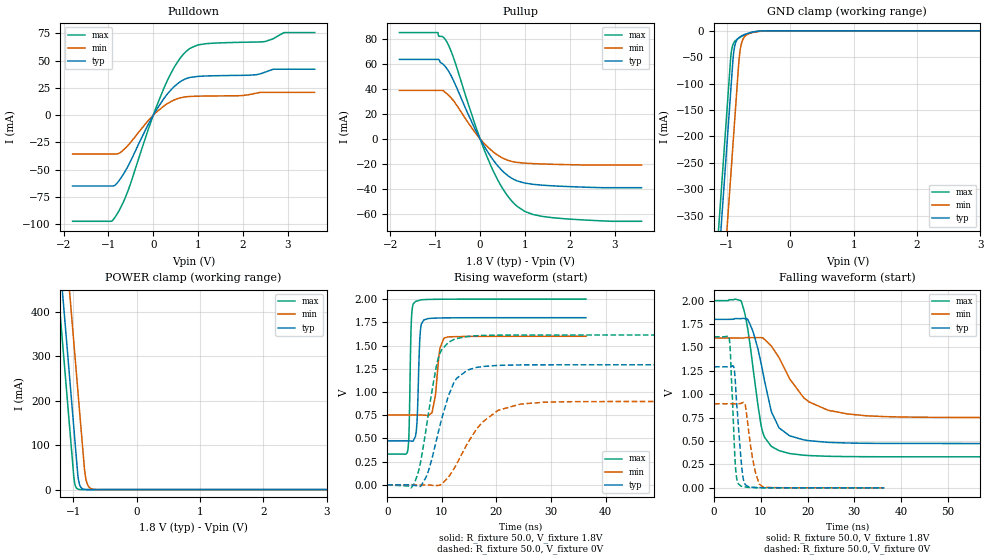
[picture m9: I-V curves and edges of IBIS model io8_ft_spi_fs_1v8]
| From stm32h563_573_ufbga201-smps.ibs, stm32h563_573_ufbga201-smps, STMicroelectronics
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[Model]   io8_ft_spi_fs_1v8
Model_type I/O
Polarity   Non-Inverting
Enable   Active-Low
| CAP_THRESHOLD on pad IOFT is "UDTCAPC" :
| Rising=20.0% of vddiom   Falling=80.0% of vddiom
| C_comp min and max val. don't necessarily correlate with the min and max pvt
| but are the smallest and greatest pad capacitance found.
| var   typ   min   max
C_comp   4.56197pF  4.45395pF  4.75009pF
|C_comp_pullup   2.85165pF  2.67170pF  2.77185pF
|C_comp_pulldown   1.71032pF  1.78225pF  1.97824pF
Vinl = 480.0mV
Vinh = 1.4V
Vmeas = 900.0mV   | Reference voltage for timing measurements
Cref  = 50.0pF   | Timing specification test load capacitance value
Rref  = 100.0MOhm   | Timing specification test load resistance value
Vref  = 900.0mV   | Timing specification test load voltage
[Model Spec]
| TIME_THRESHOLD on pin ZIV11 is "CMOS" :
| Rising=40.0% of vdd   Falling=60.0% of vdd
Vinl 703.80000mV 631.80000mV 784.80000mV
Vinh 1.06220V 937.20000mV 1.16620V
| variable   typ   min   max
[Temperature Range] 25.0 125.0 -40.0
| variable   typ   min   max
[Voltage Range] 1.8V 1.6V 2.0V
| variable   typ   min   max
[POWER Clamp Reference] 1.8V 1.6V 2.0V
| variable   typ   min   max
[GND Clamp Reference] 0V 0V 0V
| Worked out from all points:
|   slope of the pulldown table from 0 to 0.27 V, typ, clamps not added: 15.8 ohm
|   slope of the pullup table from 0 to 0.27 V, typ, clamps not added: 17.1 ohm
|   GND clamp passes 1 mA (typ) near -0.52 V on its own axis
|   POWER clamp passes 1 mA (typ) near -0.84 V on its own axis
|   rising waveform, R_fixture 50.0, V_fixture 1.8V: 20-80 % time 436ps typ, 865ps min, 327ps max; typ from 0.474 V to 1.8 V
|   falling waveform, R_fixture 50.0, V_fixture 1.8V: 20-80 % time 3.87ns typ, 6.87ns min, 2.77ns max; typ from 1.8 V to 0.474 V
|   rising waveform, R_fixture 50.0, V_fixture 0V: 20-80 % time 3.66ns typ, 6.11ns min, 2.71ns max; typ from 0 V to 1.29 V
|   falling waveform, R_fixture 50.0, V_fixture 0V: 20-80 % time 1.19ns typ, 1.67ns min, 840ps max; typ from 1.29 V to 0 V
[POWER Clamp]
-1.8V     1.518A     1.709A     1.407A
-1.23V    548.8mA    740.2mA    437.5mA
-1.16V    429.8mA    621.2mA    318.5mA
-1.05V    242.8mA    434.2mA    131.5mA
-980mV    123.8mA    315.2mA    17.95mA
-930mV    38.81mA    230.2mA    1.49mA
-910mV    17.82mA    196.2mA    550.8uA
-890mV    8.18mA     162.2mA    203.5uA
-810mV    363.5uA    33.6mA     3.797uA
-770mV    76.62uA    10.47mA    518.8nA
-710mV    7.417uA    1.822mA    26.38nA
3.6V      0A         0A         0A
[GND Clamp]
-1.8V     -1.581A    -1.742A    -1.516A
-1.24V    -628.8mA   -789.9mA   -564.1mA
-1.05V    -305.8mA   -466.9mA   -241.1mA
-940mV    -118.8mA   -279.9mA   -54.1mA
-930mV    -101.8mA   -262.9mA   -41.86mA
-900mV    -51.51mA   -211.9mA   -25.34mA
-880mV    -32.22mA   -177.9mA   -21mA
-810mV    -13.02mA   -59.5mA    -13.82mA
-770mV    -9.8mA     -24.99mA   -11mA
-680mV    -5.275mA   -7.288mA   -5.917mA
-400mV    -107uA     -349.1uA   -42.51uA
3.6V      5.392nA    968.2nA    261.3pA
| variable   typ   min   max
[Pullup Reference] 1.8V 1.6V 2.0V
| variable   typ   min   max
[Pulldown Reference] 0V 0V 0V
[Pullup]
-1.8V     63.43mA    38.65mA    84.86mA
-940mV    63.43mA    38.65mA    84.86mA
-930mV    63.43mA    38.65mA    82.78mA
-770mV    57.47mA    36.83mA    79.08mA
-600mV    47.06mA    30.74mA    65.48mA
-120mV    8.364mA    5.386mA    12.19mA
240mV     -14.24mA   -8.79mA    -21.45mA
540mV     -26.97mA   -15.94mA   -41.71mA
830mV     -33.6mA    -18.8mA    -53.95mA
1.18V     -36.29mA   -19.75mA   -60.37mA
1.56V     -37.38mA   -20.24mA   -62.7mA
3.6V      -38.97mA   -20.89mA   -65.81mA
[Pulldown]
-1.8V     -65.02mA   -35.56mA   -97.42mA
-940mV    -65.02mA   -35.56mA   -97.42mA
-850mV    -64.17mA   -35.56mA   -93.5mA
-570mV    -47.32mA   -28.01mA   -70.04mA
-120mV    -9.088mA   -5.279mA   -14.07mA
250mV     16.04mA    8.832mA    26.05mA
550mV     29.17mA    15.25mA    49.41mA
780mV     34.17mA    17.07mA    60.14mA
1.18V     35.97mA    17.56mA    65.65mA
2.49V     39.44mA    20.93mA    67.53mA
2.92V     42.19mA    20.93mA    75.82mA
3.6V      42.19mA    20.93mA    75.82mA
[Ramp]
dV/dt_r 775.81477mV/3.60386ns 538.94493mV/5.87876ns 968.32434mV/2.70601ns
dV/dt_f 795.78719mV/3.67646ns 508.98073mV/6.78614ns 1.00099V/2.77286ns
R_load = 50.0
| Removed startup time: 0s 0s 0s  .
| Removed end time: 36.4ns.
[Rising Waveform]
R_fixture   = 50.0
V_fixture   = 1.8V
V_fixture_min = 1.6V
V_fixture_max = 2.0V
0s        473.7mV    751.7mV    331.7mV
3.75ns    473.7mV    751.7mV    370.1mV
4ns       473.6mV    751.7mV    599.1mV
4.45ns    471.4mV    751.7mV    1.808V
5.15ns    518.9mV    751.7mV    1.974V
6.05ns    1.645V     751.8mV    1.99V
6.7ns     1.776V     751.2mV    1.995V
8.2ns     1.794V     777.7mV    1.998V
10.4ns    1.798V     1.581V     1.999V
36.4ns    1.8V       1.6V       2V
| Removed startup time: 0s 0s 0s  .
| Removed end time: 199.4ns.
[Falling Waveform]
R_fixture   = 50.0
V_fixture   = 1.8V
V_fixture_min = 1.6V
V_fixture_max = 2.0V
0s        1.8V       1.6V       2V
5.8ns     1.808V     1.6V       1.994V
6.85ns    1.804V     1.605V     1.798V
8.15ns    1.692V     1.604V     1.357V
10.5ns    1.221V     1.599V     580.4mV
12.3ns    809.2mV    1.512V     441.7mV
16.3ns    554.2mV    1.155V     365.8mV
24.4ns    486mV      828.8mV    337.1mV
36.65ns   474.7mV    760.8mV    332.1mV
199.4ns   473.7mV    751.7mV    331.7mV
| Removed startup time: 0s 0s 0s  .
| Removed end time: 199.3ns.
[Rising Waveform]
R_fixture   = 50.0
V_fixture   = 0V
V_fixture_min = 0V
V_fixture_max = 0V
0s        134.8nV    547.1nV    93.88nV
4.4ns     178.4uV    1.8uV      -29.25mV
6.2ns     -8.613mV   17.32uV    277.3mV
7.6ns     161mV      -733.5uV   790.4mV
9.6ns     626.6mV    -2.816mV   1.408V
12.2ns    1.1V       170.8mV    1.565V
14.7ns    1.236V     448.5mV    1.598V
20.3ns    1.287V     803mV      1.612V
28.5ns    1.293V     889.3mV    1.614V
199.3ns   1.293V     898.2mV    1.614V
| Removed startup time: 0s 0s 0s  .
| Removed end time: 36.4ns.
[Falling Waveform]
R_fixture   = 50.0
V_fixture   = 0V
V_fixture_min = 0V
V_fixture_max = 0V
0s        1.293V     898.3mV    1.614V
3.25ns    1.293V     898.3mV    1.595V
4.3ns     1.271V     898.3mV    497.7mV
4.65ns    1.05V      898.2mV    179.4mV
5.2ns     657.7mV    897.9mV    43.26mV
5.95ns    208.9mV    906.4mV    16.12mV
6.55ns    45.96mV    903.7mV    10.66mV
8.55ns    5.519mV    234.5mV    2.295mV
10.4ns    2.124mV    11.95mV    980.8uV
36.4ns    4.498uV    29.17uV    3.34uV
